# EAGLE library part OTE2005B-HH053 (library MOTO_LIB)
+/- 5V charge pump
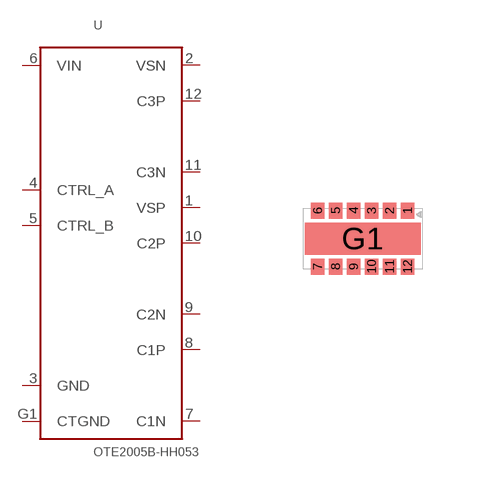
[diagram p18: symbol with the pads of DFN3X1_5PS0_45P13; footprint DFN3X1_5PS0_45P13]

Designator prefix U

## OTE2005B-HH053 (MPN: OTE2005BHH053; SUPPLIER: ORISE)  [DFN3X1_5PS0_45P13]
1  VSP
2  VSN
3  GND
4  CTRL_A
5  CTRL_B
6  VIN
7  C1N
8  C1P
9  C2N
10  C2P
11  C3N
12  C3P
G1  CTGND

## Footprint DFN3X1_5PS0_45P13 (pad centres in mm)
smd 0.33 x 0.4: 1 1.125,0.7; 2 0.675,0.7; 3 0.225,0.7; 4 -0.225,0.7; 5 -0.675,0.7; 6 -1.125,0.7; 7 -1.125,-0.7; 8 -0.675,-0.7; 9 -0.225,-0.7; 10 0.225,-0.7; 11 0.675,-0.7; 12 1.125,-0.7
smd 2.9 x 0.8: G1 0,0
